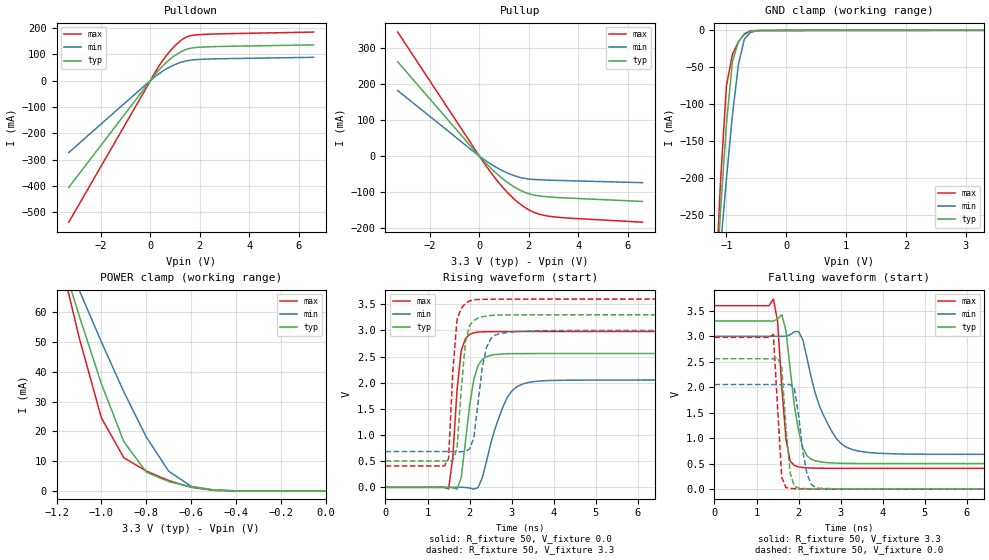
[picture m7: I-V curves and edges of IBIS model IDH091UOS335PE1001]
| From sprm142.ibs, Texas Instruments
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[Model]   IDH091UOS335PE1001
| I/O with pulldown
Model_type   I/O
Vinh = 2.00
Vinl = 0.80
Enable   Active-Low
Polarity   Non-Inverting
| signals   A, GZ, Y
Vmeas = 1.5
|   typ   min   max
C_comp   3.034p   3.016p   3.1959p
|   typ   min   max
[Temperature Range]   25   -40   125
|   typ   min   max
[Voltage Range]   3.30V   3.00V   3.60V
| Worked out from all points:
|   slope of the pulldown table from 0 to 0.495 V, typ, clamps not added: 8.97 ohm
|   slope of the pullup table from 0 to 0.495 V, typ, clamps not added: 13.9 ohm
|   GND clamp passes 1 mA (typ) near -0.59 V on its own axis
|   POWER clamp passes 1 mA (typ) near -0.57 V on its own axis
|   rising waveform, R_fixture 50, V_fixture 0.0: 20-80 % time 250ps typ, 477ps min, 168ps max; typ from 0 V to 2.56 V
|   falling waveform, R_fixture 50, V_fixture 3.3: 20-80 % time 275ps typ, 573ps min, 167ps max; typ from 3.3 V to 0.503 V
|   rising waveform, R_fixture 50, V_fixture 3.3: 20-80 % time 167ps typ, 235ps min, 145ps max; typ from 0.503 V to 3.3 V
|   falling waveform, R_fixture 50, V_fixture 0.0: 20-80 % time 149ps typ, 212ps min, 128ps max; typ from 2.56 V to 0 V
[Pulldown]
|   Voltage   I(typ)   I(min)   I(max)
-3.3V     -405.5mA   -273.2mA   -537.5mA
300mV     35.25mA    22.75mA    48.21mA
600mV     64.95mA    41.72mA    89.2mA
800mV     81.64mA    52.25mA    112.5mA
1.2V      107.5mA    68.13mA    149.4mA
1.5V      119.8mA    75.48mA    166.9mA
2V        126.6mA    80.41mA    174.4mA
6.6V      135.3mA    88.27mA    184mA
[GND_clamp]
|   Voltage   I(typ)   I(min)   I(max)
-3.3V     -3.491A    -2.631A    -4.527A
-1.2V     -379.5mA   -393.3mA   -377.9mA
-1.1V     -246.8mA   -295.2mA   -206.6mA
-1V       -126.7mA   -201.3mA   -75.29mA
-900mV    -42.19mA   -115.1mA   -32.37mA
-800mV    -14.98mA   -46.32mA   -15.54mA
-700mV    -5.444mA   -11.69mA   -4.594mA
-600mV    -1.095mA   -2.791mA   -595uA
-500mV    -140.5uA   -516.3uA   -93.45uA
-400mV    -41.27uA   -80.01uA   -55.76uA
3.3V      100.3uA    56.21uA    176.6uA
[Pullup]
|   Voltage   I(typ)   I(min)   I(max)
-3.3V     261.2mA    181.5mA    343.6mA
-200mV    15.59mA    10.64mA    20.79mA
300mV     -22.18mA   -14.8mA    -30.05mA
700mV     -48.7mA    -32mA      -66.54mA
1V        -66mA      -42.81mA   -90.87mA
1.3V      -80.83mA   -51.65mA   -112.3mA
1.6V      -92.95mA   -58.38mA   -130.4mA
1.9V      -102.1mA   -62.82mA   -145.1mA
2.2V      -108.1mA   -65mA      -155.8mA
2.8V      -113.3mA   -66.81mA   -166.6mA
3.6V      -116.6mA   -68.38mA   -172mA
6.6V      -125.9mA   -73.9mA    -183.4mA
[POWER_clamp]
|   Voltage   I(typ)   I(min)   I(max)
-3.3V     641.5mA    488.2mA    827.1mA
-1.2V     83.53mA    85.64mA    83.49mA
-1.1V     59.03mA    67.58mA    51.73mA
-1V       35.97mA    50mA       24.51mA
-900mV    16.54mA    33.24mA    11.13mA
-800mV    6.31mA     18.09mA    6.679mA
-700mV    3.132mA    6.592mA    3.469mA
-600mV    1.316mA    1.559mA    1.222mA
-500mV    313uA      327.2uA    181.3uA
-400mV    30.67uA    45.43uA    9.59uA
0V        1pA        1pA        1pA
[Ramp]
|   I(typ)   I(min)   I(max)
dV/dt_r   1.536/0.242n   1.231/0.470n   1.788/0.155n
dV/dt_f   1.678/0.267n   1.390/0.572n   1.915/0.163n
[Rising Waveform]
R_fixture = 50
V_fixture = 0.0
|  pu_on
|  TIME   V(typ)   V(min)   V(max)
0s        3nV        14nV       2nV
1.5ns     1.614mV    315.1uV    -29.5mV
1.6ns     -8.483mV   626uV      580.1mV
1.7ns     -33.57mV   1.061mV    1.856V
1.8ns     189mV      1.25mV     2.616V
2.1ns     2.063V     -34.84mV   2.956V
2.3ns     2.444V     183.7mV    2.973V
2.9ns     2.553V     1.728V     2.979V
3.3ns     2.557V     1.986V     2.979V
10ns      2.559V     2.052V     2.98V
[Falling Waveform]
R_fixture = 50
V_fixture = 3.3
V_fixture_min = 3.0
V_fixture_max = 3.6
|  pd_on
|  TIME   V(typ)   V(min)   V(max)
0s        3.3V       3V         3.6V
1.4ns     3.298V     3V         3.731V
1.5ns     3.338V     2.999V     3.302V
1.6ns     3.424V     2.998V     2.011V
1.7ns     3.113V     3.001V     981.8mV
1.9ns     1.64V      3.092V     465.7mV
2.2ns     654.4mV    2.568V     418.3mV
2.6ns     526.9mV    1.438V     410.5mV
3.2ns     506mV      800.3mV    408.7mV
10ns      502.8mV    684.1mV    408.3mV
[Rising Waveform]
R_fixture = 50
V_fixture = 3.3
V_fixture_min = 3.0
V_fixture_max = 3.6
|  pd_off
|  TIME   V(typ)   V(min)   V(max)
0s        502.8mV    683.6mV    408.3mV
1.5ns     503.4mV    684.2mV    551.4mV
1.6ns     512.3mV    684.2mV    2.217V
1.7ns     739.2mV    683.6mV    3.207V
1.9ns     2.78V      686.8mV    3.517V
2ns       3.097V     734.8mV    3.565V
2.1ns     3.191V     950.4mV    3.585V
2.4ns     3.277V     2.674V     3.596V
2.6ns     3.291V     2.908V     3.598V
10ns      3.3V       3V         3.6V
[Falling Waveform]
R_fixture = 50
V_fixture = 0.0
|  pu_off
|  TIME   V(typ)   V(min)   V(max)
0s        2.559V     2.053V     2.98V
1.4ns     2.558V     2.052V     3.036V
1.6ns     2.39V      2.051V     230.8mV
1.7ns     1.214V     2.054V     31.12mV
1.8ns     311.9mV    2.054V     15.23mV
1.9ns     52.85mV    1.971V     8.821mV
2.1ns     13.44mV    740mV      3.739mV
2.2ns     8.973mV    300.1mV    2.726mV
2.4ns     4.81mV     32.44mV    1.558mV
10ns      349nV      98.77uV    5.934uV
